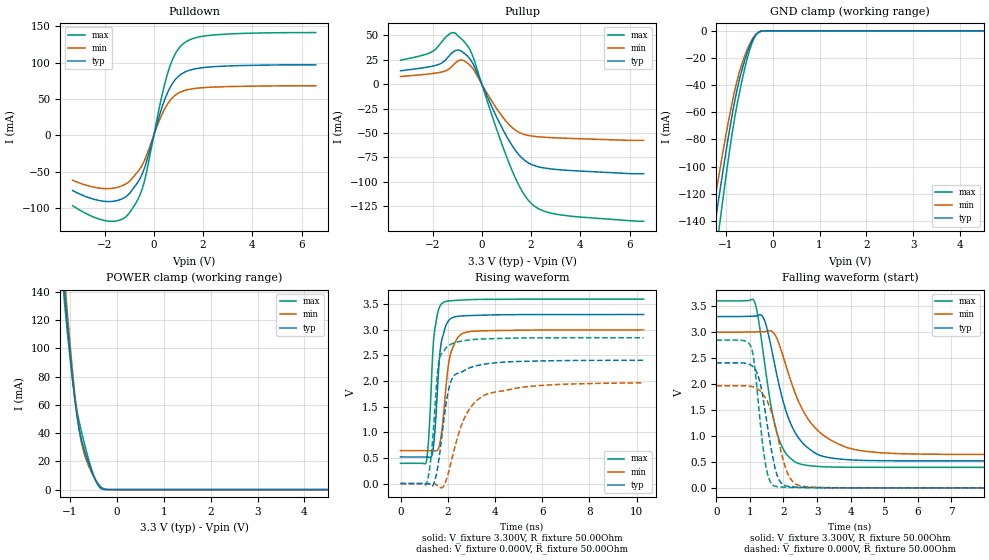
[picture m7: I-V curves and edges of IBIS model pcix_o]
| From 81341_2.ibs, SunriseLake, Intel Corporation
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[Model]   pcix_o
Model_type   Output
|Vinl = 1.155V
|Vinh = 1.650V
Vmeas = 1.320V
Vref = 0.000V
Cref = 10.000pF
Rref = 100.000Ohm
|   typ   min   max
C_comp   7.500pF   6.000pF   9.000pF
[Voltage Range]   3.300V   3.000V   3.600V
[Temperature Range]   60.0   110.0   -5.0
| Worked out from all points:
|   slope of the pulldown table from 0 to 0.495 V, typ, clamps not added: 9.23 ohm
|   slope of the pullup table from 0 to 0.495 V, typ, clamps not added: 17.7 ohm
|   GND clamp passes 1 mA (typ) near -0.29 V on its own axis
|   POWER clamp passes 1 mA (typ) near -0.32 V on its own axis
|   falling waveform, V_fixture 3.300V, R_fixture 50.00Ohm: 20-80 % time 716ps typ, 1.02ns min, 495ps max; typ from 3.3 V to 0.519 V
|   rising waveform, V_fixture 3.300V, R_fixture 50.00Ohm: 20-80 % time 260ps typ, 348ps min, 224ps max; typ from 0.519 V to 3.3 V
|   rising waveform, V_fixture 0.000V, R_fixture 50.00Ohm: 20-80 % time 459ps typ, 999ps min, 287ps max; typ from 0 V to 2.41 V
|   falling waveform, V_fixture 0.000V, R_fixture 50.00Ohm: 20-80 % time 379ps typ, 474ps min, 282ps max; typ from 2.41 V to 0 V
[Pulldown]
|   Voltage   I(typ)   I(min)   I(max)
-3.3V     -75.86mA   -61.73mA   -96.63mA
-1.85V    -90.94mA   -73.19mA   -117.8mA
-1.35V    -88.05mA   -70.09mA   -116mA
-950mV    -78.24mA   -61.8mA    -104.6mA
-600mV    -61.61mA   -47.72mA   -84.62mA
-400mV    -46.75mA   -35.92mA   -65.11mA
300mV     35.28mA    26.51mA    50.26mA
600mV     61.73mA    45.2mA     89.48mA
900mV     77.73mA    55.81mA    113.8mA
1.25V     86.75mA    61.53mA    127.2mA
2.6V      94.61mA    66.5mA     138.3mA
6.575V    96.84mA    68.07mA    141.1mA
[GND Clamp]
|   Voltage   I(typ)   I(min)   I(max)
-3.3V     -632.9mA   -564.7mA   -726mA
-1.325V   -165.7mA   -144.5mA   -196.2mA
-1.3V     -159.6mA   -139.1mA   -189.2mA
-1.25V    -147.7mA   -128.5mA   -175.4mA
-1.2V     -135.9mA   -118mA     -161.8mA
-1.125V   -118.5mA   -102.6mA   -141.6mA
-850mV    -59.68mA   -50.83mA   -73.04mA
-650mV    -28.43mA   -23.95mA   -36.35mA
-450mV    -8.224mA   -7.115mA   -10.15mA
-350mV    -2.584mA   -2.414mA   -2.804mA
-250mV    -331.4uA   -398.2uA   -220.5uA
6.575V    0A         0A         0A
[Pullup]
|   Voltage   I(typ)   I(min)   I(max)
-3.3V     13.6mA     7.765mA    24.4mA
-2.15V    17.57mA    10.35mA    31.46mA
-1.75V    20.06mA    11.71mA    39.24mA
-1.35V    28.16mA    15.15mA    50.46mA
-1.1V     33.87mA    20.89mA    52.24mA
-800mV    33.19mA    24.5mA     45.58mA
-400mV    22.59mA    17.05mA    30.81mA
1.1V      -57.44mA   -41.16mA   -80.22mA
1.6V      -74.74mA   -50.3mA    -107.8mA
2V        -81.94mA   -52.96mA   -121.7mA
3.05V     -87.28mA   -55mA      -133mA
6.575V    -91.64mA   -57.46mA   -140.2mA
[POWER Clamp]
|   Voltage   I(typ)   I(min)   I(max)
-3.3V     1.119A     1.097A     1.143A
-1.125V   145.9mA    154.5mA    136.9mA
-1.1V     135.7mA    144.2mA    127.5mA
-1.05V    116.3mA    124mA      110.3mA
-900mV    65.35mA    69.46mA    66.19mA
-800mV    42.32mA    42.13mA    47.87mA
-750mV    34.9mA     32.74mA    40.7mA
-650mV    23.68mA    21.07mA    27.47mA
-500mV    10.21mA    9.628mA    10.7mA
-400mV    3.805mA    4.129mA    3.114mA
-300mV    590.7uA    960.3uA    205.7uA
6.575V    0A         0A         0A
[Ramp]
R_load = 50.00Ohm
|   typ   min   max
dV/dt_r   1.444V/458.811ps   1.180V/998.346ps   1.708V/287.180ps
dV/dt_f   1.668V/715.489ps   1.414V/1.015ns   1.923V/495.145ps
[Falling Waveform]
V_fixture = 3.300V
V_fixture_min = 3.000V
V_fixture_max = 3.600V
R_fixture = 50.00Ohm
|   Time   V(typ)   V(min)   V(max)
0s        3.3V       3V         3.6V
1.13ns    3.307V     3.004V     3.596V
1.24ns    3.322V     3.005V     3.306V
1.44ns    3.221V     3.008V     2.395V
1.77ns    2.276V     2.922V     1.142V
2.06ns    1.511V     2.384V     675.3mV
2.38ns    1.029V     1.77V      487.1mV
3.04ns    636.1mV    1.094V     412mV
4.12ns    534.9mV    738mV      396.4mV
10.3ns    519.4mV    642.6mV    394.8mV
[Rising Waveform]
V_fixture = 3.300V
V_fixture_min = 3.000V
V_fixture_max = 3.600V
R_fixture = 50.00Ohm
|   Time   V(typ)   V(min)   V(max)
0s        519.4mV    642.6mV    394.8mV
1.08ns    519.4mV    642.3mV    404.7mV
1.2ns     515.7mV    642.4mV    934.8mV
1.33ns    551.6mV    642.6mV    2.204V
1.42ns    834.3mV    641.3mV    2.893V
1.65ns    2.448V     750.2mV    3.443V
1.79ns    2.875V     1.196V     3.528V
2.09ns    3.206V     2.476V     3.567V
2.63ns    3.273V     2.93V      3.582V
10.3ns    3.3V       3V         3.6V
[Rising Waveform]
V_fixture = 0.000V
V_fixture_min = 0.000V
V_fixture_max = 0.000V
R_fixture = 50.00Ohm
|   Time   V(typ)   V(min)   V(max)
0s        524.1nV    3.8uV      30.23nV
1.1ns     92.97uV    -257.7uV   -7.214mV
1.3ns     -41.25mV   43.88uV    550.2mV
1.44ns    37.87mV    -2.832mV   1.368V
1.62ns    449.7mV    -59.04mV   2.376V
1.83ns    1.221V     -45.41mV   2.579V
2.07ns    1.893V     284.1mV    2.703V
2.71ns    2.209V     1.282V     2.791V
3.63ns    2.336V     1.739V     2.824V
10.3ns    2.406V     1.967V     2.846V
[Falling Waveform]
V_fixture = 0.000V
V_fixture_min = 0.000V
V_fixture_max = 0.000V
R_fixture = 50.00Ohm
|   Time   V(typ)   V(min)   V(max)
0s        2.406V     1.967V     2.846V
1.04ns    2.36V      1.953V     2.705V
1.14ns    2.3V       1.933V     2.357V
1.26ns    2.129V     1.89V      1.584V
1.45ns    1.496V     1.746V     514.2mV
1.72ns    467.9mV    1.283V     38.86mV
1.88ns    141.3mV    838.5mV    18.23mV
2.1ns     33.58mV    314.5mV    10.16mV
2.53ns    9.959mV    35.18mV    3.789mV
10.3ns    524.1nV    3.8uV      30.23nV
